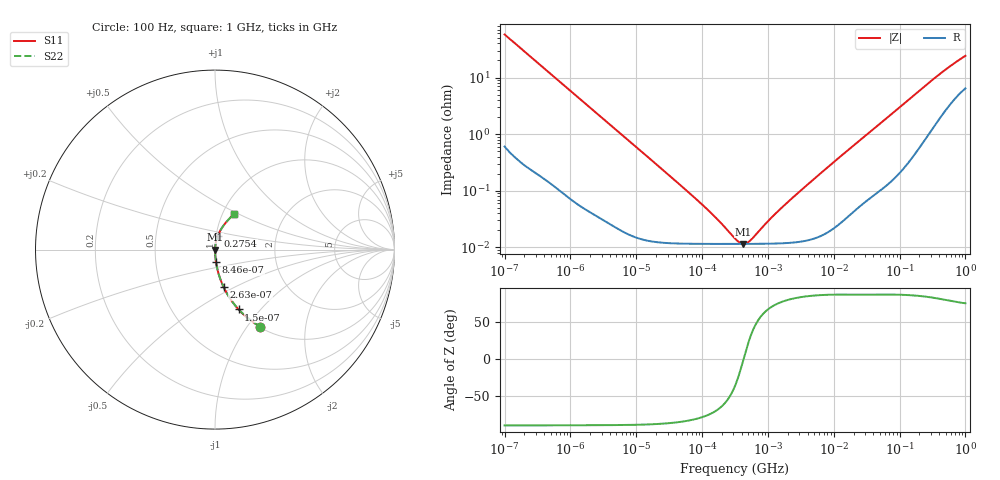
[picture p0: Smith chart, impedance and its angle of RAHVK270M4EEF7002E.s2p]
! RAHVK270M4EEF7002E  S-PARAMETER MODEL  (AEC-Q200 qualified)
! Model Generated by ELNA Corporation (http://www.ty-top.com)
! Version 1.0
! ELNA Control No. 201214
! Copyright (c) 2020 ELNA CO.,LTD. All Rights Reserved.
! Products Name : CONDUCTIVE POLYMER HYBRID ALUMINUM ELECTROLYTIC CAPACITORS
! Characteristics :
!  Capacitance  :  27uF  ,  Rated voltage  :  63V
!  Operating Temp. Range  :  -55 to +125 degC  ,  Endurance  :  4000hr at 125 degC
!  Dimension D  :  8mm  ,  Dimension L  :  8.7mm
! Frequency Range : 100Hz - 1GHz
! External Node Assignments :
!  1  o---| |---o  2
# MHz S RI R 50
!Freq[MHz].  S11 Real  S11 Imag  S21 Real  S21 Imag  S12 Real  S12 Imag  S22 Real  S22 Imag
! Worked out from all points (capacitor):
!   401 points, 100 Hz to 1 GHz, reference 50 ohm
!   read as one part in series: C = 27.6 uF near 108 Hz
!   lowest |Z| = 11.5 mohm at 419.3 kHz (marker M1)
!   series resonance near 427.9 kHz, so ESL is about 5 nH
!   S11 on the Smith chart (normalised r, x): 100 Hz: 1.01, -1.15; 150 Hz: 1.01, -0.77; 263 Hz: 1.00, -0.44; 846 Hz: 1.00, -0.14; 275.4 MHz: 1.02, +0.16; 1 GHz: 1.13, +0.47
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0.0001  0.2516 -0.4287  0.7484 0.4287  0.7484 0.4287  0.2516 -0.4287
0.00015  0.1317 -0.3334  0.8683 0.3334  0.8683 0.3334  0.1317 -0.3334
0.000198  0.0802 -0.2668  0.9198 0.2668  0.9198 0.2668  0.0802 -0.2668
0.000263  0.048 -0.2087  0.952 0.2087  0.952 0.2087  0.048 -0.2087
0.000462  0.0169 -0.1231  0.9831 0.1231  0.9831 0.1231  0.0169 -0.1231
0.000846  0.00553 -0.0684  0.9945 0.0684  0.9945 0.0684  0.00553 -0.0684
0.001488  0.00205 -0.0392  0.9979 0.0392  0.9979 0.0392  0.00205 -0.0392
0.004241  0.000439 -0.0139  0.9996 0.0139  0.9996 0.0139  0.000439 -0.0139
0.022131  0.00013 -0.00267  0.9999 0.00267  0.9999 0.00267  0.00013 -0.00267
0.120226  0.000116 -0.000454  0.9999 0.000454  0.9999 0.000454  0.000116 -0.000454
0.187284  0.000115 -0.000256  0.9999 0.000256  0.9999 0.000256  0.000115 -0.000256
0.316228  0.000115 -8.51e-05  0.9999 8.51e-05  0.9999 8.51e-05  0.000115 -8.51e-05
0.371535  0.000115 -3.92e-05  0.9999 3.92e-05  0.9999 3.92e-05  0.000115 -3.92e-05
0.419276  0.000115 -5.58e-06  0.9999 5.58e-06  0.9999 5.58e-06  0.000115 -5.58e-06
0.473151  0.000115 2.8e-05  0.9999 -2.8e-05  0.9999 -2.8e-05  0.000115 2.8e-05
0.555904  0.000115 7.35e-05  0.9999 -7.35e-05  0.9999 -7.35e-05  0.000115 7.35e-05
1.348963  0.000117 0.000393  0.9999 -0.000393  0.9999 -0.000393  0.000117 0.000393
4.704354  0.000142 0.00151  0.9999 -0.00151  0.9999 -0.00151  0.000142 0.00151
69.9842  0.0018 0.0209  0.9982 -0.0209  0.9982 -0.0209  0.0018 0.0209
275.4229  0.0158 0.0774  0.9842 -0.0774  0.9842 -0.0774  0.0158 0.0774
568.8529  0.0514 0.1391  0.9486 -0.1391  0.9486 -0.1391  0.0514 0.1391
1000  0.1035 0.1966  0.8965 -0.1966  0.8965 -0.1966  0.1035 0.1966
